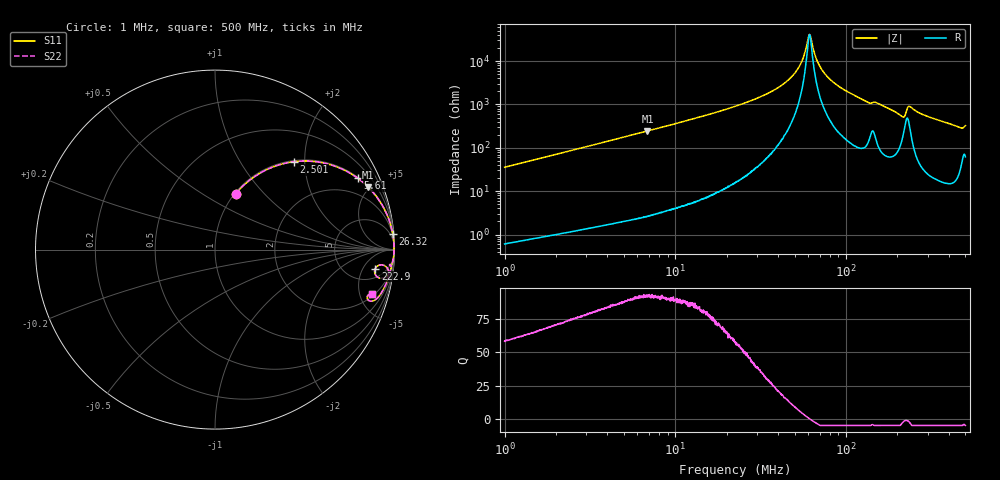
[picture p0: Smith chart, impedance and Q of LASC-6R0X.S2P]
!s-Parameter Generated by FASTRON Sdn. Bhd.
!FASTRON P/N : LASC-6R0X
!Keysight Technologies,E4991B,MY54100416,A.01.15
!Date: Tue Mar 17 09:53:40 2026
!Version  : Rev00 Tue Mar 17 09:53:40 2026
!Data & Calibration Information:
!PortZ  Port1:50+j0  Port2:50+j0
!When reading, reference impedance value at option line is always used.
! Remarks : This data is being provided solely for informational purposes.
!Freq	S11	S21	S12	S22
# Hz S dB R 50
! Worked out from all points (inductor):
!   1601 points, 1 MHz to 500 MHz, reference 50 ohm
!   read as one part in series: L = 5.64 uH near 1.032 MHz
!   highest Q = 92.7 at 6.866 MHz (marker M1), where L = 5.65 uH
!   self-resonance near 61.15 MHz
!   S11 on the Smith chart (normalised r, x): 1 MHz: 1.01, +0.71; 2.501 MHz: 1.02, +1.76; 5.61 MHz: 1.04, +3.97; 26.32 MHz: 1, +23; 222.9 MHz: 8, -9; 500 MHz: 2.24, -6.36
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1000000  -9.55 69.6  -0.56 -19.4  -0.56 -19.4  -9.55 69.6
2500910  -3.64 48.1  -2.56 -41.1  -2.56 -41.1  -3.64 48.1
2820919  -3.09 44.8  -3.04 -44.5  -3.04 -44.5  -3.09 44.8
5610017  -1.02 26.6  -6.97 -62.7  -6.97 -62.7  -1.02 26.6
6865635  -0.71 22.2  -8.44 -67.2  -8.44 -67.2  -0.71 22.2
7957584  -0.54 19.4  -9.59 -70.0  -9.59 -70.0  -0.54 19.4
2.236068e7  -0.07 6.3  -19.17 -82.7  -19.17 -82.7  -0.07 6.3
2.632285e7  -0.05 5.1  -21.10 -83.8  -21.10 -83.8  -0.05 5.1
4.605113e7  -0.02 1.5  -31.40 -84.1  -31.40 -84.1  -0.02 1.5
5.400095e7  -0.02 0.7  -38.49 -78.7  -38.49 -78.7  -0.02 0.7
6.043941e7  -0.02 0.1  -51.50 -25.7  -51.50 -25.7  -0.02 0.1
6.307767e7  -0.02 -0.2  -48.52 49.6  -48.52 49.6  -0.02 -0.2
7.005203e7  -0.02 -0.7  -37.70 77.4  -37.70 77.4  -0.02 -0.7
8.343135e7  -0.03 -1.7  -30.52 82.5  -30.52 82.5  -0.03 -1.7
1.329695e8  -0.11 -4.9  -21.25 79.1  -21.25 79.1  -0.11 -4.9
1.77937e8  -0.15 -7.0  -18.26 78.6  -18.26 78.6  -0.15 -7.0
2.119214e8  -0.56 -9.8  -15.03 64.4  -15.03 64.4  -0.56 -9.8
2.228968e8  -0.92 -6.8  -16.43 44.7  -16.43 44.7  -0.92 -6.8
2.36269e8  -0.35 -5.8  -19.40 65.3  -19.40 65.3  -0.35 -5.8
3.23625e8  -0.26 -11.7  -13.83 75.8  -13.83 75.8  -0.26 -11.7
4.62629e8  -0.72 -18.2  -10.08 66.4  -10.08 66.4  -0.72 -18.2
5e8  -0.84 -16.0  -11.05 63.0  -11.05 63.0  -0.84 -16.0
